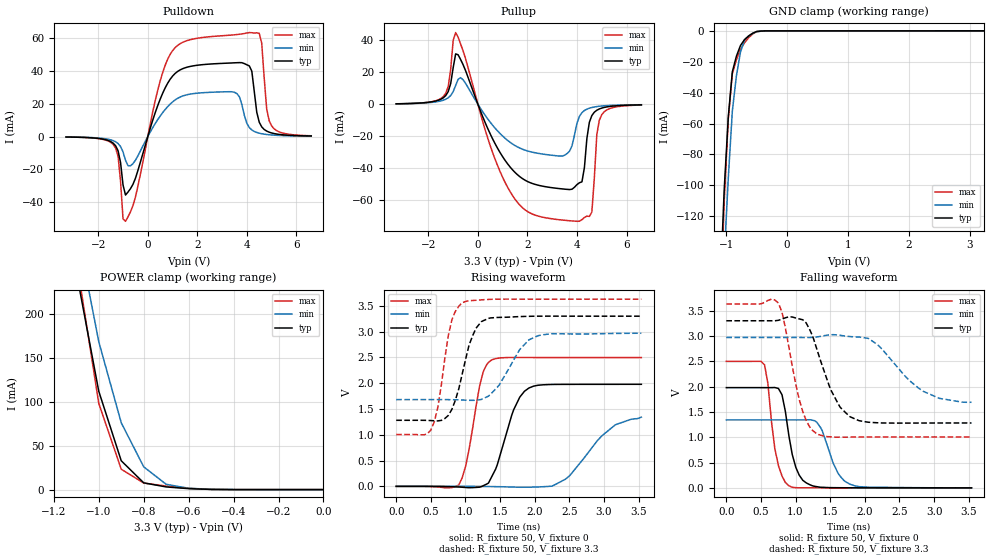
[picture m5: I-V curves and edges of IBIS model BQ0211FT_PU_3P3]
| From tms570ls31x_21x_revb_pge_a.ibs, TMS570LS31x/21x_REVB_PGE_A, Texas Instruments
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|   Model Cell BQ0211FT_PU_3P3
|BQ0211FT_PU_3P3
[Model]   BQ0211FT_PU_3P3
Model_type   I/O
Polarity   Non-Inverting
Enable   Active-Low
Vinl =  1.15
Vinh =  1.55
Cref =  15.0001pF
Rref =  101.0000M
Vref =  0V
Vmeas =  1.65
C_comp   1.2p   1.2p   1.2p
[Model Spec]
Vinl   1.15   1.02   1.28
Vinh   1.55   1.45   1.65
[Temperature Range]   25   155   -40
[Voltage Range]   3.3   2.97   3.63
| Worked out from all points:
|   slope of the pulldown table from 0 to 0.495 V, typ, clamps not added: 22 ohm
|   slope of the pullup table from 0 to 0.495 V, typ, clamps not added: 26.9 ohm
|   GND clamp passes 1 mA (typ) near -0.53 V on its own axis
|   POWER clamp passes 1 mA (typ) near -0.59 V on its own axis
|   rising waveform, R_fixture 50, V_fixture 0: 20-80 % time 279ps typ, 513ps min, 195ps max; typ from 0 V to 1.98 V
|   rising waveform, R_fixture 50, V_fixture 3.3: 20-80 % time 240ps typ, 354ps min, 183ps max; typ from 1.28 V to 3.3 V
|   falling waveform, R_fixture 50, V_fixture 0: 20-80 % time 164ps typ, 225ps min, 138ps max; typ from 1.98 V to 0.001 V
|   falling waveform, R_fixture 50, V_fixture 3.3: 20-80 % time 335ps typ, 537ps min, 238ps max; typ from 3.3 V to 1.28 V
[POWER_clamp]
|   voltage   I(typ)   I(min)   I(max)
-3.3V     4.054A     4.63A      4.887A
-1.1V     248.3mA    301mA      262.7mA
-1.067V   202.9mA    256.9mA    207.9mA
-1.033V   157.5mA    212.7mA    153.1mA
-1V       112.1mA    168.6mA    98.31mA
-900mV    32.89mA    76.23mA    23.24mA
-800mV    7.72mA     25.95mA    7.497mA
-700mV    3.046mA    6.046mA    4.01mA
-600mV    1.099mA    1.535mA    1.442mA
-500mV    196.6uA    374.7uA    217.1uA
0V        442.7pA    6.158nA    416.6pA
[Pulldown]
|   voltage   I(typ)   I(min)   I(max)
-3.3V     -289uA     -253.9uA   -287.1uA
-1.4V     -4mA       -2.489mA   -4.76mA
-1.2V     -8.69mA    -4.261mA   -12.05mA
-1V       -29.49mA   -9.376mA   -50.19mA
-900mV    -35.6mA    -14.42mA   -51.59mA
1V        36.78mA    21.07mA    52.28mA
3.5V      44.86mA    26.91mA    61.93mA
4.1V      42.98mA    5.455mA    63.29mA
4.6V      5.887mA    1.718mA    56.92mA
4.8V      3.323mA    1.257mA    16.92mA
5V        2.171mA    957.9uA    6.458mA
6.6V      331.3uA    239.5uA    466.8uA
[Pullup]
|   voltage   I(typ)   I(min)   I(max)
-3.3V     325.3uA    297.6uA    301.6uA
-1.4V     4.042mA    2.556mA    4.795mA
-1.2V     7.932mA    4.062mA    11.12mA
-900mV    31.45mA    11.76mA    44.76mA
1.4V      -40.91mA   -24.77mA   -56.99mA
3.4V      -52.76mA   -32.29mA   -72.18mA
4V        -50.08mA   -11.8mA    -72.98mA
4.2V      -48.37mA   -5.201mA   -71.98mA
4.6V      -7.019mA   -1.989mA   -67.23mA
4.8V      -3.708mA   -1.414mA   -19.03mA
5V        -2.349mA   -1.055mA   -6.475mA
6.6V      -340.9uA   -258.1uA   -448.7uA
[GND_clamp]
|   voltage   I(typ)   I(min)   I(max)
-3.3V     -3.25A     -2.875A    -4.945A
-1.1V     -166.9mA   -205.1mA   -187mA
-1.033V   -102.8mA   -146.7mA   -110.1mA
-966.7mV  -55.96mA   -95.69mA   -57.02mA
-900mV    -26.55mA   -52.03mA   -27.8mA
-833.3mV  -16.5mA    -29.28mA   -18.78mA
-766.7mV  -9.55mA    -13.91mA   -12.09mA
-700mV    -5.706mA   -5.929mA   -7.734mA
-566.7mV  -1.585mA   -1.639mA   -2.086mA
-500mV    -421.6uA   -604.2uA   -492.4uA
-366.7mV  -38.21uA   -69.49uA   -50.21uA
3.233V    -1.13uA    7.006uA    -9.303uA
[Ramp]
| variable   typ   min   max
dV/dt_f   1.259958/0.3442833n  0.8120091/0.5599962n   1.637516/0.2457655n
dV/dt_r   1.203363/0.2797725n  0.8165906/0.5189591n   1.517779/0.1975198n
R_load = 50
[Rising Waveform]
R_fixture = 50
V_fixture = 0
V_fixture_min = 0
V_fixture_max = 0
|   time   V(typ)   V(min)   V(max)
0s        260.7uV    208.4uV    321uV
904ps     -12.36mV   406.5uV    27.57mV
1.004ns   -21.68mV   462.7uV    399.8mV
1.256ns   12.62mV    -1.617mV   2.219V
1.384ns   199.7mV    -4.115mV   2.455V
1.696ns   1.485V     -13.67mV   2.499V
1.916ns   1.907V     -16.39mV   2.498V
2.444ns   1.978V     140mV      2.497V
3.164ns   1.979V     1.193V     2.498V
3.54ns    1.979V     1.342V     2.498V
[Rising Waveform]
R_fixture = 50
V_fixture = 3.3
V_fixture_min = 2.97
V_fixture_max = 3.63
|   time   V(typ)   V(min)   V(max)
0s        1.281V     1.682V     1.006V
500ps     1.276V     1.682V     1.093V
600ps     1.27V      1.682V     1.529V
804ps     1.493V     1.681V     3.23V
952ps     2.173V     1.675V     3.561V
1.152ns   3.066V     1.671V     3.608V
1.332ns   3.256V     1.749V     3.625V
1.784ns   3.292V     2.654V     3.63V
2.048ns   3.3V       2.921V     3.63V
3.54ns    3.3V       2.969V     3.63V
[Falling Waveform]
R_fixture = 50
V_fixture = 0
V_fixture_min = 0
V_fixture_max = 0
|   time   V(typ)   V(min)   V(max)
0s        1.98V      1.342V     2.498V
552ps     1.979V     1.342V     2.429V
700ps     1.982V     1.342V     777.6mV
804ps     1.839V     1.342V     235mV
904ps     1.023V     1.342V     41.6mV
1.052ns   252.4mV    1.342V     764.8uV
1.256ns   35.81mV    1.332V     1.009mV
1.616ns   3.16mV     282.9mV    750.8uV
1.784ns   1.768mV    73.39mV    784.7uV
3.54ns    549.1uV    736.5uV    348.9uV
[Falling Waveform]
R_fixture = 50
V_fixture = 3.3
V_fixture_min = 2.97
V_fixture_max = 3.63
|   time   V(typ)   V(min)   V(max)
0s        3.3V       2.97V      3.63V
752ps     3.309V     2.97V      3.649V
804ps     3.332V     2.97V      3.467V
1.104ns   3.319V     2.97V      1.506V
1.308ns   2.735V     2.98V      1.064V
1.512ns   1.927V     3.023V     1.007V
1.784ns   1.406V     2.988V     1.003V
2.18ns    1.286V     2.832V     1.006V
2.84ns    1.28V      1.909V     1.007V
3.54ns    1.282V     1.69V      1.007V
